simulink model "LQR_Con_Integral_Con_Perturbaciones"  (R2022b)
settings: Solver=ode4  StartTime=0.0  StopTime=0.2  FixedStep=1e-6  RelTol=1e-3
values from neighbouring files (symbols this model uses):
  A = [-R_1/L_1,  omega_1    [LQR_Con_Integral.m]    (also in PI_Lazo_V_DC.m = -10000; LQR_Sin_Integral.m; Modal_Integral.m)
  B = [-V_DC0/(2*L_1*m_t1),  0    [LQR_Con_Integral.m]    (also in PI_Lazo_V_DC.m = 10000; LQR_Sin_Integral.m; Modal_Integral.m)
  C = eye(2)    [LQR_Con_Integral.m]    (also in PI_Lazo_V_DC.m = 1; LQR_Sin_Integral.m; Modal_Integral.m)
  D = zeros(2)    [LQR_Con_Integral.m]    (also in PI_Lazo_V_DC.m = 0; LQR_Sin_Integral.m; Modal_Integral.m)
  E = [1/L_1,  0    [LQR_Con_Integral.m]    (also in LQR_Sin_Integral.m; Modal_Integral.m)
  Kc = Kca(:, 1:2)    [LQR_Con_Integral.m]    (also in Modal_Integral.m = Kca_place(:, 1:2))
  Ki = -Kca(:, 3:4)    [LQR_Con_Integral.m]    (also in Modal_Integral.m = -Kca_place(:, 3:4))
  tau = te    (= 0.001)    [LQR_Con_Integral.m]    (also in IP_Lazo_P_2.m = 0.002; IP_Lazo_Q_12.m = 0.002; LQR_Sin_Integral.m = 0.002; Modal_Integral.m)
  v_d_1 = 100*sqrt(2)    [LQR_Con_Integral.m]    (also in PI_Lazo_V_DC.m; LQR_Sin_Integral.m; Modal_Integral.m; Sistema_no_lineal_Modal.m)
  v_q_1 = 0    [LQR_Con_Integral.m]    (also in LQR_Sin_Integral.m; Modal_Integral.m)

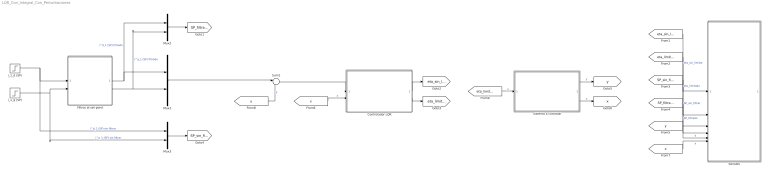
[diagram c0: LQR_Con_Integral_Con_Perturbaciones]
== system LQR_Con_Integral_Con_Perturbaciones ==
  Controlador LQR : Subsystem
  Filtros al set-point : Subsystem
  Mux1 : Mux  Inputs=2
  Mux2 : Mux  Inputs=2
  Mux3 : Mux  Inputs=2
  Señales : Subsystem
  Sistema a controlar : Subsystem
  Sum1 : Sum  Inputs=|+-
  i_1_d (SP) : Step  Time=0.05  Before=18  After=-2  SampleTime=0
  i_1_q (SP) : Step  Time=0.05  Before=-15  After=-5  SampleTime=0
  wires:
  Mux2/1 -> [SP_filtrado]
  Sistema a controlar/1(y) -> [y]  "y"
  Sistema a controlar/2(x) -> [x]  "x"
  i_1_d (SP)/1 -> Mux3/1, Filtros al set-point/1(i_1_d sin filtrar)  "i^d_1 (SP) sin filtrar"
  i_1_q (SP)/1 -> Mux3/2, Filtros al set-point/2(i_1_q sin filtrar)  "i^q_1 (SP) sin filtrar"
  Mux3/1 -> [SP_sin_filtrar]
  [eta_sin_limitar] -> Señales/1(eta_sin_limitar)  "eta_sin_limitar"
  [eta_limitado] -> Señales/2(eta_limitado)  "eta_limitado"
  [SP_sin_filtrar] -> Señales/3(SP_sin_filtrar)  "SP_sin_filtrar"
  [SP_filtrado] -> Señales/4(SP_filtrado)  "SP_filtrado"
  [y] -> Señales/5(y)  "y"
  [x] -> Señales/6(x)  "x"
  Filtros al set-point/1(i_1_d filtrado) -> Mux2/1, Mux1/1  "i^d_1 (SP) filtrado"
  Filtros al set-point/2(i_1_q filtrado) -> Mux1/2, Mux2/2  "i^q_1 (SP) filtrado"
  [y] -> Sum1/2  "y"
  Controlador LQR/2(eta limitado) -> [eta_limitado]
  Sum1/1 -> Controlador LQR/1(e)
  Controlador LQR/1(eta sin limitar) -> [eta_sin_limitar]
  [x] -> Controlador LQR/2(x)  "x"
  [eta_limitado] -> Sistema a controlar/1(u)  "u"
  Mux1/1 -> Sum1/1

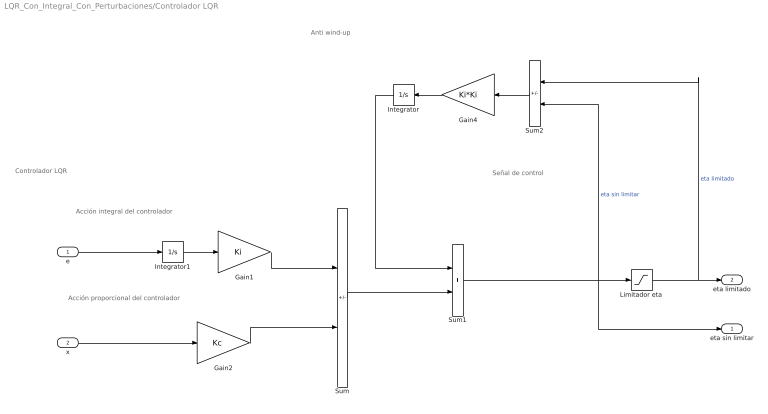
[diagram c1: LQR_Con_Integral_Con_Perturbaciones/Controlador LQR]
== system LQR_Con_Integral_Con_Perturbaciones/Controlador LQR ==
  note: Señal de control
  note: Anti wind-up
  note: Controlador LQR
  note: Acción proporcional del controlador
  note: Acción integral del controlador
  e : Inport
  x : Inport  Port=2
  Gain1 : Gain  Gain=Ki  Multiplication=Matrix(K*u) (u vector)
  Gain2 : Gain  Gain=Kc  Multiplication=Matrix(K*u) (u vector)
  Gain4 : Gain  Gain=Ki*Ki  Multiplication=Matrix(K*u) (u vector)
  Integrator : Integrator
  Integrator1 : Integrator
  Limitador eta : Saturate  UpperLimit=5  LowerLimit=-5
  Sum : Sum  Inputs=+-
  Sum1 : Sum
  Sum2 : Sum  Inputs=+-
  eta sin limitar : Outport
  eta limitado : Outport  Port=2
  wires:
  Gain1/1 -> Sum/1
  x/1 -> Gain2/1
  Gain2/1 -> Sum/2
  Limitador eta/1 -> eta limitado/1, Sum2/1  "eta limitado"
  e/1 -> Integrator1/1
  Integrator/1 -> Sum1/1
  Sum2/1 -> Gain4/1
  Sum1/1 -> eta sin limitar/1, Sum2/2, Limitador eta/1  "eta sin limitar"
  Gain4/1 -> Integrator/1
  Integrator1/1 -> Gain1/1
  Sum/1 -> Sum1/2

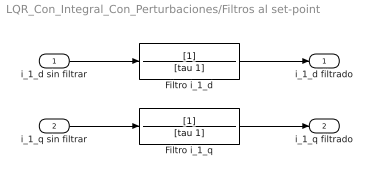
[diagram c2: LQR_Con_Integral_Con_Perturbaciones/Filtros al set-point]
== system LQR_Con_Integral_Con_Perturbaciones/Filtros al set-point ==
  i_1_d sin filtrar : Inport
  i_1_q sin filtrar : Inport  Port=2
  Filtro i_1_d : TransferFcn  Denominator=[tau 1]
  Filtro i_1_q : TransferFcn  Denominator=[tau 1]
  i_1_d filtrado : Outport
  i_1_q filtrado : Outport  Port=2
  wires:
  i_1_q sin filtrar/1 -> Filtro i_1_q/1
  i_1_d sin filtrar/1 -> Filtro i_1_d/1
  Filtro i_1_d/1 -> i_1_d filtrado/1
  Filtro i_1_q/1 -> i_1_q filtrado/1

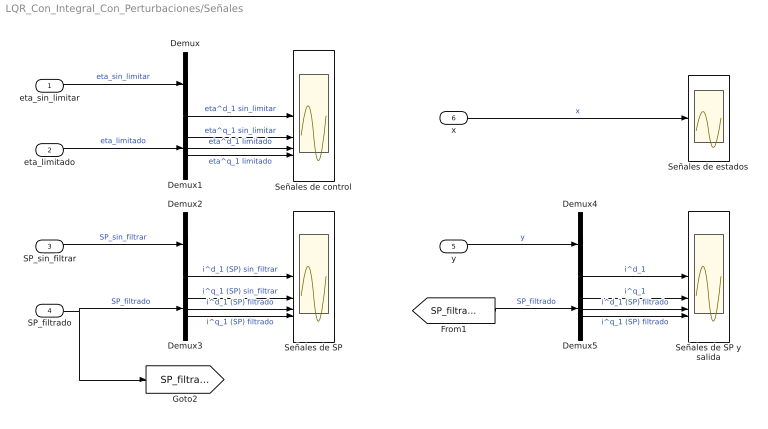
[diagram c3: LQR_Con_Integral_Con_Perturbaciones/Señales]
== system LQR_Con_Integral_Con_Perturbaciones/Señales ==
  eta_sin_limitar : Inport
  eta_limitado : Inport  Port=2
  SP_sin_filtrar : Inport  Port=3
  SP_filtrado : Inport  Port=4
  y : Inport  Port=5
  x : Inport  Port=6
  Demux{,1..5} (6 alike) : Demux  Outputs=2
  Señales de SP : Scope  NumInputPorts=4
  Señales de SP y salida : Scope  NumInputPorts=4
  Señales de control : Scope  NumInputPorts=4
  Señales de estados : Scope
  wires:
  y/1 -> Demux4/1  "y"
  eta_sin_limitar/1 -> Demux/1  "eta_sin_limitar"
  SP_filtrado/1 -> [SP_filtrado], Demux3/1  "SP_filtrado"
  x/1 -> Señales de estados/1  "x"
  SP_sin_filtrar/1 -> Demux2/1  "SP_sin_filtrar"
  eta_limitado/1 -> Demux1/1  "eta_limitado"
  [SP_filtrado] -> Demux5/1  "SP_filtrado"
  Demux1/2 -> Señales de control/4  "eta^q_1 limitado"
  Demux/1 -> Señales de control/1  "eta^d_1 sin_limitar"
  Demux/2 -> Señales de control/2  "eta^q_1 sin_limitar"
  Demux1/1 -> Señales de control/3  "eta^d_1 limitado"
  Demux3/1 -> Señales de SP/3  "i^d_1 (SP) filtrado"
  Demux3/2 -> Señales de SP/4  "i^q_1 (SP) filtrado"
  Demux2/2 -> Señales de SP/2  "i^q_1 (SP) sin_filtrar"
  Demux2/1 -> Señales de SP/1  "i^d_1 (SP) sin_filtrar"
  Demux4/1 -> Señales de SP y salida/1  "i^d_1"
  Demux4/2 -> Señales de SP y salida/2  "i^q_1"
  Demux5/2 -> Señales de SP y salida/4  "i^q_1 (SP) filtrado"
  Demux5/1 -> Señales de SP y salida/3  "i^d_1 (SP) filtrado"

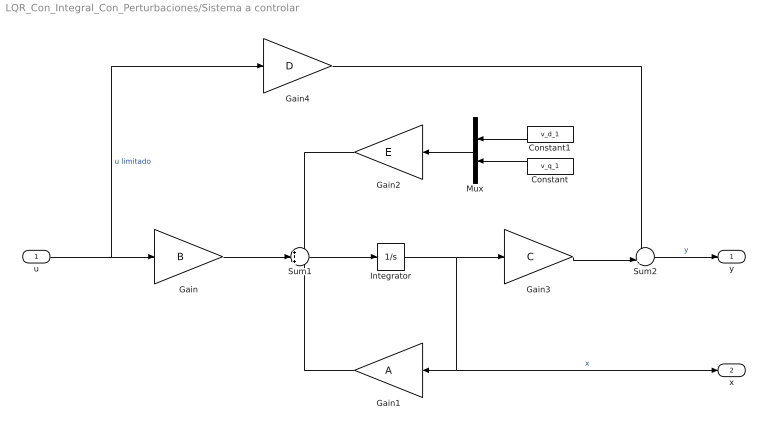
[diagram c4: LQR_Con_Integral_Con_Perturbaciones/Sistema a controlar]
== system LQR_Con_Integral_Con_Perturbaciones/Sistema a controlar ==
  u : Inport
  Constant : Constant  Value=v_q_1
  Constant1 : Constant  Value=v_d_1
  Gain : Gain  Gain=B  Multiplication=Matrix(K*u) (u vector)
  Gain1 : Gain  Gain=A  Multiplication=Matrix(K*u) (u vector)
  Gain2 : Gain  Gain=E  Multiplication=Matrix(K*u) (u vector)
  Gain3 : Gain  Gain=C  Multiplication=Matrix(K*u) (u vector)
  Gain4 : Gain  Gain=D  Multiplication=Matrix(K*u) (u vector)
  Integrator : Integrator
  Mux : Mux  Inputs=2
  Sum1 : Sum  Inputs=+++
  Sum2 : Sum  Inputs=++|
  y : Outport
  x : Outport  Port=2
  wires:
  Gain/1 -> Sum1/2
  Gain1/1 -> Sum1/3
  Integrator/1 -> x/1, Gain1/1, Gain3/1  "x"
  Sum2/1 -> y/1  "y"
  Sum1/1 -> Integrator/1
  Gain3/1 -> Sum2/2
  Gain4/1 -> Sum2/1
  u/1 -> Gain4/1, Gain/1  "u limitado"
  Mux/1 -> Gain2/1
  Constant1/1 -> Mux/1
  Constant/1 -> Mux/2
  Gain2/1 -> Sum1/1
